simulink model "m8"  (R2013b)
settings: Solver=ode45  StartTime=0.0  StopTime=50  RelTol=1e-3
undefined symbols (not defined in the file): dend, DiscIntNeverNeededParam, Ki, Kp, numd, Tlim, Ts
libraries: powerlib x46, simulink x5, powerlib_extras x3

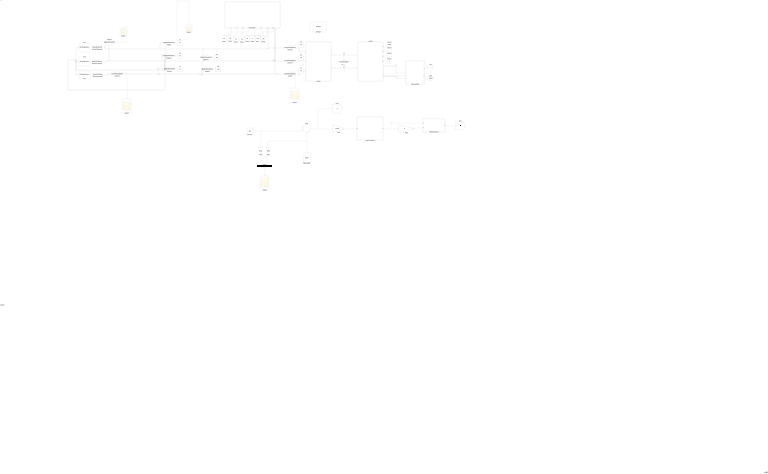
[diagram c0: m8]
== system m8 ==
  AC4 : powerlib/Electrical Sources/AC Voltage Source  Amplitude=400  Phase=0  Frequency=50  SampleTime=0  Measurements=None
  AC5 : powerlib/Electrical Sources/AC Voltage Source  Amplitude=400  Phase=120  Frequency=50  SampleTime=0  Measurements=None
  AC6 : powerlib/Electrical Sources/AC Voltage Source  Amplitude=400  Phase=240  Frequency=50  SampleTime=0  Measurements=None
  Bus Creator : BusCreator  Inputs=2
  C1 : powerlib/Elements/Series RLC Branch  LConnTagsString=__new0  RConnTagsString=__new0  BranchType=C  Resistance=1  Inductance=1e-3  SetiL0=off  InitialCurrent=0  Capacitance=50e-2  Setx0=off  InitialVoltage=0  Measurements=None
  Constant : Constant  Value=146
  Current {,1..3} (4 alike) : powerlib/Measurements/Current Measurement  PhasorSimulation=off  OutputType=Complex  PSBequivalent=0
  Gain3 : Gain  Gain=30/pi
  Gain4 : Gain  Gain=30/pi
  Gain5 : Gain  Gain=8
  Gain6 : Gain  Gain=1/(2*pi)
  Induction Motor : Subsystem
  Integrator : Integrator
  MATLAB Function1 : MATLAB Function  TreatAsAtomicUnit=on
  Mux1 : Mux  Inputs=2
  Scope{1..4,9} (5 alike) : Scope
  Series RLC Branch3 : powerlib/Elements/Series RLC Branch  LConnTagsString=__new0  RConnTagsString=__new0  BranchType=RL  Resistance=0.025  Inductance=80e-6  SetiL0=off  InitialCurrent=0  Capacitance=1e-6  Setx0=off  InitialVoltage=0  Measurements=None
  Series RLC Branch5 : powerlib/Elements/Series RLC Branch  LConnTagsString=__new0  RConnTagsString=__new0  BranchType=RL  Resistance=0.025  Inductance=80e-6  SetiL0=off  InitialCurrent=0  Capacitance=1e-6  Setx0=off  InitialVoltage=0  Measurements=None
  Series RLC Branch7 : powerlib/Elements/Series RLC Branch  LConnTagsString=__new0  RConnTagsString=__new0  BranchType=RL  Resistance=0.025  Inductance=80e-6  SetiL0=off  InitialCurrent=0  Capacitance=1e-6  Setx0=off  InitialVoltage=0  Measurements=None
  Speed controller2 : Subsystem
  Sum4 : Sum  Inputs=|+-
  Voltage {,1..5} (6 alike) : powerlib/Measurements/Voltage Measurement  PhasorSimulation=off  OutputType=Complex  PSBequivalent=0
  inverter : Subsystem
  powergui : powerlib/powergui  Priority=1  SimulationMode=Discrete  SolverType=Tustin  SampleTime=50e-6  frequency=60  SPID=off  DisableSnubberDevices=off  DisableRonSwitches=off  DisableVfSwitches=off  SwTol=0  Interpol=off  DisplayEquations=off  frequencyindice=0  Pbase=100e6  ErrMax=1e-4  Iterations=50  UnitsV=kV  UnitsW=MW  FunctionMessages=off  echomessages=off  HookPort=off  EnableUseOfTLC=off  x0status=blocks  RestoreLinks=warning  ResistiveCurrentMeasurement=off  Frange=[0:2:500]  Ylog=off  Xlog=on  ShowGrid=off  save=off  variable=ZData  structure=ScopeData5  ZoomFFT=off  StartTime=9.8  cycles=1  DisplayStyle=1  fundamental=50  FreqAxis=on  MaxFrequency=1000  frequencyindicesteady=1  RmsSteady=1  display=off  Ts=0  methode=off
  rectifire : Subsystem
  shunt filter : Subsystem
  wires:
  Mux1/1 -> Scope9/1
  [speed] -> inverter/1(speed)
  Sum4/1 -> [e], Gain6/1
  [speed] -> Gain4/1, Sum4/2
  Induction Motor/1(iabc) -> [i]
  Induction Motor/2(speed(rad/s)) -> [speed]
  [i] -> inverter/2(iabc)
  Speed controller2/1(f*) -> Gain5/1, MATLAB Function1/1(f)
  Gain5/1 -> MATLAB Function1/2(v)
  MATLAB Function1/1(Fi) -> [Fi]
  [e] -> inverter/4(e(Te))
  Gain3/1 -> Mux1/1
  Gain4/1 -> Mux1/2
  Gain6/1 -> Speed controller2/1(e)
  [Fi] -> inverter/3(phir*)
  [iLa] -> shunt filter/1(iLa)
  [iLb] -> shunt filter/2(iLb)
  [iLc] -> shunt filter/3(iLc)
  "Voltage "/1 -> Scope1/1, [va]
  Voltage 1/1 -> [vb]
  Voltage 2/1 -> [vc]
  [va] -> shunt filter/4(va)
  [vb] -> shunt filter/5(vb)
  [vc] -> shunt filter/6(vc)
  Voltage 3/1 -> Scope2/1
  [vab] -> shunt filter/7(vab)
  [vcb] -> shunt filter/8(vcb)
  "Current "/1 -> Scope3/1, [iLc]
  Current 2/1 -> [iLa]
  Current 1/1 -> [iLb]
  Voltage 4/1 -> [vab]
  Voltage 5/1 -> [vcb]
  Constant/1 -> Gain3/1, Sum4/1
  Current 3/1 -> Scope4/1
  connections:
  C1/LConn1 -- rectifire/RConn1 -- inverter/RConn1
  C1/RConn1 -- inverter/RConn2 -- rectifire/RConn2
  Voltage 2/LConn2 -- AC5/LConn1 -- AC6/LConn1 -- AC4/LConn1 -- "Voltage "/LConn2 -- Voltage 1/LConn2
  shunt filter/LConn3 -- "Current "/LConn1 -- Voltage 5/LConn1 -- Voltage 2/LConn1 -- Current 3/RConn1
  "Voltage "/LConn1 -- Voltage 3/LConn1 -- Series RLC Branch3/RConn1 -- Voltage 4/LConn1 -- shunt filter/LConn1 -- Current 2/LConn1
  shunt filter/LConn2 -- Current 1/LConn1 -- Voltage 4/LConn2 -- Voltage 5/LConn2 -- Voltage 3/LConn2 -- Series RLC Branch5/RConn1 -- Voltage 1/LConn1
  inverter/LConn1 -- Induction Motor/LConn1
  inverter/LConn2 -- Induction Motor/LConn2
  Series RLC Branch3/LConn1 -- AC4/RConn1
  Series RLC Branch7/LConn1 -- AC6/RConn1
  inverter/LConn3 -- Induction Motor/LConn3
  Series RLC Branch5/LConn1 -- AC5/RConn1
  Current 2/RConn1 -- rectifire/LConn1
  Current 1/RConn1 -- rectifire/LConn2
  "Current "/RConn1 -- rectifire/LConn3
  Series RLC Branch7/RConn1 -- Current 3/LConn1

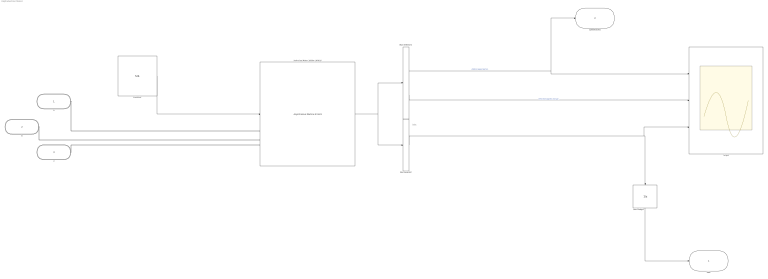
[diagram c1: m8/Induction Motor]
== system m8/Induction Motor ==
  note: iabc
  Bus Selector : BusSelector  OutputSignals=Stator measurements.Stator current is_a (A),Stator measurements.Stator current is_b (A),Stator measurements.Stator current is_c (A)  OutputAsBus=on
  Bus Selector1 : BusSelector  OutputSignals=Mechanical.Rotor speed (wm),Mechanical.Electromagnetic torque Te (N*m)
  Constant : Constant  Value=526
  Induction Motor 100kw / 400 V : powerlib/Machines/Asynchronous Machine SI Units  PresetModel=No  MechanicalLoad=Torque Tm  ShowDetailedParameters=on  RotorType=Squirrel-cage  ReferenceFrame=Rotor  NominalParameters=[ 100e3, 400, 50 ]  Stator=[ 0.087 0.8e-3 ]  Rotor="[ 0.228  0.8e-3 ]"  Cage1=[ 0.022 0.226/377]  Cage2=[ 0.022 0.226/377]  Lm=34.7e-3  Mechanical="[0.3  0.1 2 ]"  PolePairs=2  InitialConditions="[ 1, 0 ,  0 , 0 , 0 , 0 , 0 , 0 ]"  Units=SI  LoadFlowParameters=0  SimulateSaturation=off  Saturation=[0 0;0 0]  TsPowergui=0  TsBlock=-1  IterativeModel=Trapezoidal non iterative  Pmec=0
  Scope : Scope  NumInputPorts=3
  Unit Delay4 : UnitDelay  SampleTime=50e-6
  a : PMIOPort  Port=1  Side=Left
  b : PMIOPort  Port=2  Side=Left
  " c" : PMIOPort  Port=3  Side=Left
  iabc : Outport
  speed(rad/s) : Outport  Port=2
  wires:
  Bus Selector1/1 -> speed(rad/s)/1, Scope/1  "<Rotor speed (wm)>"
  Induction Motor 100kw / 400 V/1 -> Bus Selector1/1, Bus Selector/1
  Bus Selector1/2 -> Scope/2  "<Electromagnetic torque Te (N*m)>"
  Bus Selector/1 -> Unit Delay4/1, Scope/3
  Unit Delay4/1 -> iabc/1
  Constant/1 -> Induction Motor 100kw / 400 V/1
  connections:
  " c"/RConn1 -- Induction Motor 100kw / 400 V/LConn3
  a/RConn1 -- Induction Motor 100kw / 400 V/LConn1
  b/RConn1 -- Induction Motor 100kw / 400 V/LConn2

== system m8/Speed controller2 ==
  e : Inport
  Discrete-Time Integrator : DiscreteIntegrator  IntegratorMethod=Integration: Trapezoidal  SampleTime=Ts  LimitOutput=on  UpperSaturationLimit=Tlim  LowerSaturationLimit=0  ICPrevOutput=DiscIntNeverNeededParam  ICPrevScaledInput=DiscIntNeverNeededParam
  Gain : Gain  Gain=Ki
  Gain1 : Gain  Gain=Kp
  Saturation : Saturate  UpperLimit=Tlim  LowerLimit=0
  Sum2 : Sum
  f* : Outport  InitialOutput=0
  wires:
  Gain1/1 -> Sum2/1
  Gain/1 -> Discrete-Time Integrator/1
  e/1 -> Gain/1, Gain1/1
  Discrete-Time Integrator/1 -> Sum2/2
  Sum2/1 -> Saturation/1
  Saturation/1 -> f*/1

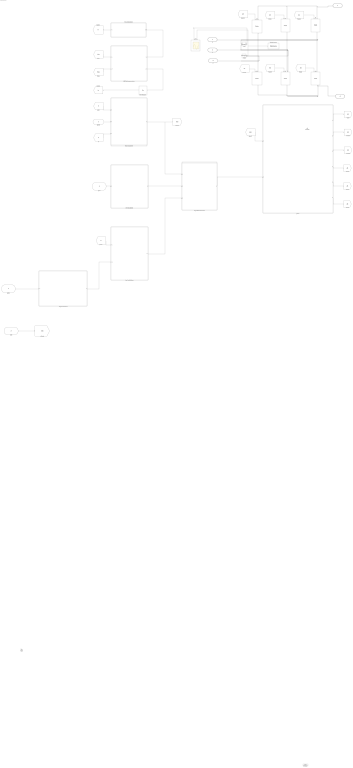
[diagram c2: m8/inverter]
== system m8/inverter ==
  speed : Inport
  iabc : Inport  Port=2
  phir* : Inport  Port=3
  e(Te) : Inport  Port=4
  ABC to dq conversion : Subsystem
  Display : Display
  Flux Calculation : Subsystem
  Gain : Gain
  S{1..6} (6 alike) : powerlib/Power Electronics/IGBT//Diode  Ron=1e-3  Rs=1e5  Cs=inf  Measurements=on
  Teta Calculation : Subsystem
  To Workspace : ToWorkspace  VariableName=VacM  SampleTime=-1  SaveFormat=Timeseries
  Torque controller : Subsystem
  Unit Delay5 : UnitDelay  SampleTime=50e-6
  Vac : powerlib/Measurements/Voltage Measurement  PhasorSimulation=off  OutputType=Complex  PSBequivalent=0
  Vac1 : powerlib/Measurements/Voltage Measurement  PhasorSimulation=off  OutputType=Complex  PSBequivalent=0
  dq to ABC conversion : Subsystem
  id* Calculation : Subsystem
  iqs* calculation : Subsystem
  pwm : Subsystem
  vac : Scope  NumInputPorts=2
  a : PMIOPort  Port=1  Side=Left
  + : PMIOPort  Port=2  Side=Right
  b : PMIOPort  Port=3  Side=Left
  _ : PMIOPort  Port=4  Side=Right
  c : PMIOPort  Port=5  Side=Left
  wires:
  [A5] -> S5/1
  [A3] -> S3/1
  [A1] -> S1/1
  [A2] -> S2/1
  [A6] -> S6/1
  [A4] -> S4/1
  Vac/1 -> vac/1
  Vac1/1 -> To Workspace/1, vac/2
  e(Te)/1 -> Torque controller/1(e)
  dq to ABC conversion/1(Iabc*) -> pwm/2(Iabc*)
  iqs* calculation/1(Iq*) -> dq to ABC conversion/3(Iq*)
  id* Calculation/1(Id*) -> dq to ABC conversion/2(Id*)
  Teta Calculation/1(Teta) -> dq to ABC conversion/1(Teta), [Teta]
  phir*/1 -> id* Calculation/1(Phir*)
  Torque controller/1(Te*) -> iqs* calculation/2(Te*)
  ABC to dq conversion/2(Iq) -> Unit Delay5/1
  ABC to dq conversion/1(Id) -> Flux Calculation/1(Id)
  Flux Calculation/1(Phir) -> [fi]
  [fi] -> Teta Calculation/1(Phir)
  Unit Delay5/1 -> [iq]
  [iq] -> Teta Calculation/3(Iq)
  [fi] -> iqs* calculation/1(Phir)
  [Teta] -> ABC to dq conversion/2(Teta)
  speed/1 -> Teta Calculation/2(wm)
  iabc/1 -> [iabc]
  [iabc] -> ABC to dq conversion/1(Iabc)
  [iabc] -> pwm/1(Iabc)
  pwm/1(s1) -> [A1]
  pwm/2(s2) -> [A2]
  pwm/3(s3) -> [A3]
  pwm/4(s4) -> [A4]
  pwm/5(s5) -> [A5]
  pwm/6(s6) -> [A6]
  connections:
  S4/RConn1 -- _/RConn1 -- S2/RConn1 -- S6/RConn1
  S6/LConn1 -- Vac1/LConn1 -- Vac/LConn2 -- b/RConn1 -- S3/RConn1
  S5/LConn1 -- S3/LConn1 -- +/RConn1 -- S1/LConn1
  S1/RConn1 -- Vac/LConn1 -- a/RConn1 -- S4/LConn1
  S5/RConn1 -- c/RConn1 -- Vac1/LConn2 -- S2/LConn1

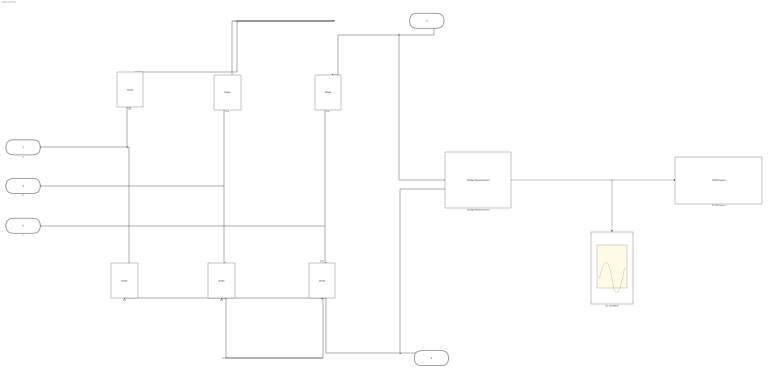
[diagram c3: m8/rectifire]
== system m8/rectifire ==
  D{1..6} (6 alike) : powerlib/Power Electronics/Diode  Ron=0.001  Lon=0  Vf=0.8  IC=0  UseSnubber=off  Rs=500  Cs=250e-9  Measurements=on
  DC VOLTAGE : Scope
  To Workspace : ToWorkspace  VariableName=VDC  SampleTime=-1  SaveFormat=Timeseries
  Voltage Measurement : powerlib/Measurements/Voltage Measurement  PhasorSimulation=off  OutputType=Complex  PSBequivalent=0
  a : PMIOPort  Port=1  Side=Left
  + : PMIOPort  Port=2  Side=Right
  b : PMIOPort  Port=3  Side=Left
  _ : PMIOPort  Port=4  Side=Right
  c : PMIOPort  Port=5  Side=Left
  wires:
  Voltage Measurement/1 -> To Workspace/1, DC VOLTAGE/1
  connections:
  Voltage Measurement/LConn2 -- _/RConn1 -- D6/LConn1 -- D4/LConn1 -- D2/LConn1
  b/RConn1 -- D6/RConn1 -- D3/LConn1
  a/RConn1 -- D4/RConn1 -- D1/LConn1
  Voltage Measurement/LConn1 -- +/RConn1 -- D1/RConn1 -- D3/RConn1 -- D5/RConn1
  c/RConn1 -- D2/RConn1 -- D5/LConn1

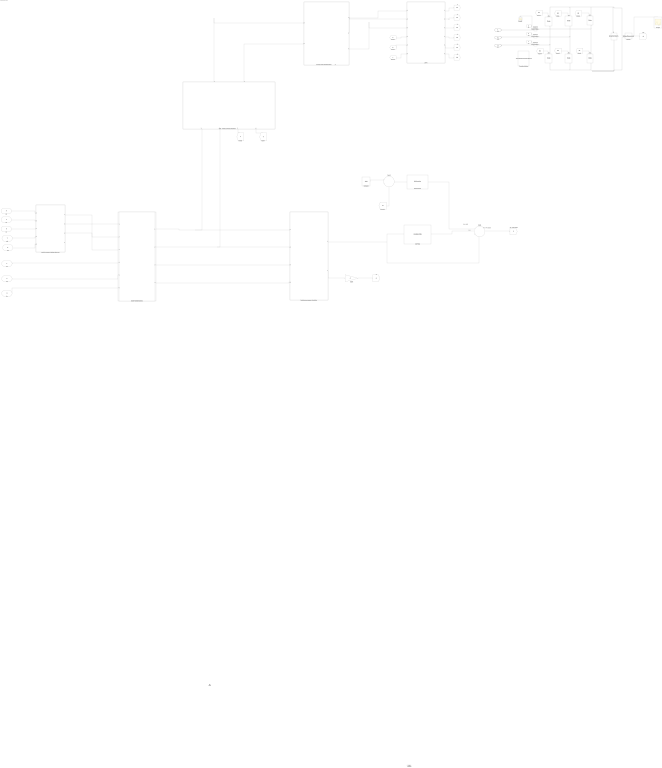
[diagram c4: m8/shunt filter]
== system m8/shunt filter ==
  note: -P(~)+P(-)LOSS
  note: P(-)
  note: P(-) LOSS
  iLa : Inport
  iLb : Inport  Port=2
  iLc : Inport  Port=3
  va : Inport  Port=4
  vb : Inport  Port=5
  vc : Inport  Port=6
  vab : Inport  Port=7
  vcb : Inport  Port=8
  " (alfa -  betta) currents calculation         " : Subsystem
  " Inverse clarke Transformation           1" : Subsystem
  2nd Filter : powerlib_extras/Control  Blocks/2nd-Order Filter  FilterType=Lowpass  Fo=50  Zeta=0.707  Initialize=off  Vac_Init=[1 45 60]  Vdc_Init=-0.5  PlotResponse=off  param1=[1 500 1]
  C : powerlib/Elements/Series RLC Branch  LConnTagsString=__new0  RConnTagsString=__new0  BranchType=C  Resistance=1  Inductance=1e-3  SetiL0=off  InitialCurrent=0  Capacitance=.045  Setx0=on  InitialVoltage=1000  Measurements=None
  Clarke Transformation1 : Subsystem
  Constant : Constant  Value=1000
  Coupling Inductor : powerlib/Elements/Three-Phase Series RLC Branch  LConnTagsString=A|B|C  RConnTagsString=A|B|C  BranchType=RL  Resistance=0.9  Inductance=0.001  Capacitance=1e-6  Measurements=None
  Current 1 : powerlib/Measurements/Current Measurement  PhasorSimulation=off  OutputType=Complex  PSBequivalent=0
  Current 2 : powerlib/Measurements/Current Measurement  PhasorSimulation=off  OutputType=Complex  PSBequivalent=0
  Current 3 : powerlib/Measurements/Current Measurement  PhasorSimulation=off  OutputType=Complex  PSBequivalent=0
  Display : Display
  Gain : Gain
  Gain6 : Gain  Gain=-1
  "Instantaneous power calculation " : Subsystem
  PID Controller : simulink/Continuous/PID Controller  Controller=PI  TimeDomain=Discrete-time  SampleTime=50e-6  IntegratorMethod=Forward Euler  FilterMethod=Forward Euler  Form=Parallel  P=400  I=100  D=0  N=100  InitialConditionSource=internal  InitialConditionForIntegrator=0  InitialConditionForFilter=0  ExternalReset=none  LimitOutput=off  UpperSaturationLimit=inf  LowerSaturationLimit=-inf  LinearizeAsGain=on  AntiWindupMode=none  Kb=1  TrackingMode=off  Kt=1  PParamMin=[]  PParamMax=[]  IParamMin=[]  IParamMax=[]  DParamMin=[]  DParamMax=[]  NParamMin=[]  NParamMax=[]  KbParamMin=[]  KbParamMax=[]  KtParamMin=[]  KtParamMax=[]  POutMin=[]  POutMax=[]  IOutMin=[]  IOutMax=[]  DOutMin=[]  DOutMax=[]  NOutMin=[]  NOutMax=[]  KbOutMin=[]  KbOutMax=[]  KtOutMin=[]  KtOutMax=[]  IntegratorOutMin=[]  IntegratorOutMax=[]  FilterOutMin=[]  FilterOutMax=[]  SumOutMin=[]  SumOutMax=[]  SumI1OutMin=[]  SumI1OutMax=[]  SumI2OutMin=[]  SumI2OutMax=[]  SumI3OutMin=[]  SumI3OutMax=[]  SumDOutMin=[]  SumDOutMax=[]  SaturationOutMin=[]  SaturationOutMax=[]  IntegratorContinuousStateAttributes=''  IntegratorStateMustResolveToSignalObject=off  IntegratorRTWStateStorageClass=Auto  FilterContinuousStateAttributes=''  FilterStateMustResolveToSignalObject=off  FilterRTWStateStorageClass=Auto
  S{1..6} (6 alike) : powerlib/Power Electronics/IGBT//Diode  Ron=1e-3  Rs=1e5  Cs=inf  Measurements=on
  Scope1 : Scope
  Scope3 : Scope
  Sum1 : Sum  Inputs=|+-
  Sum4 : Sum  Inputs=|++-
  "Voltage " : powerlib/Measurements/Voltage Measurement  PhasorSimulation=off  OutputType=Complex  PSBequivalent=0
  positive sequence Voltage Detector : Subsystem
  pwm : Subsystem
  ica : PMIOPort  Port=1  Side=Left
  icb : PMIOPort  Port=2  Side=Left
  icc : PMIOPort  Port=3  Side=Left
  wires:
  [B5] -> S5/1
  [B3] -> S3/1
  [B1] -> S1/1
  [B2] -> S2/1
  [B6] -> S6/1
  [B4] -> S4/1
  iLa/1 -> Clarke Transformation1/4(iLa)
  iLb/1 -> Clarke Transformation1/5(iLb)
  iLc/1 -> Clarke Transformation1/6(iLc)
  Clarke Transformation1/1(v alfa') -> "Instantaneous power calculation "/1(v alfa'), " (alfa -  betta) currents calculation         "/1(v alfa')
  Clarke Transformation1/2(v betta') -> "Instantaneous power calculation "/2(v betta'), " (alfa -  betta) currents calculation         "/2(v betta')
  Clarke Transformation1/3(i alfa) -> "Instantaneous power calculation "/3(i alfa)
  Clarke Transformation1/4(i betta) -> "Instantaneous power calculation "/4(i betta)
  " (alfa -  betta) currents calculation         "/1(ic alfa*) -> " Inverse clarke Transformation           1"/1(ic alfa*)
  " (alfa -  betta) currents calculation         "/2(ic betta*) -> " Inverse clarke Transformation           1"/2(ic betta*)
  "Instantaneous power calculation "/1(p) -> 2nd Filter/1, Sum4/3
  2nd Filter/1 -> Sum4/2
  PID Controller/1 -> Sum4/1
  Sum1/1 -> PID Controller/1
  Sum4/1 -> [P]
  "Instantaneous power calculation "/2(q) -> Gain6/1
  Gain6/1 -> [q]
  [P] -> " (alfa -  betta) currents calculation         "/3(-p(~)+P(-)LOSS)
  [q] -> " (alfa -  betta) currents calculation         "/4(-q)
  Current 1/1 -> [b]
  Current 2/1 -> Scope1/1, [a]
  Current 3/1 -> [c]
  [a] -> pwm/4(Ica)
  [b] -> pwm/5(Icb)
  [c] -> pwm/6(Icc)
  " Inverse clarke Transformation           1"/1(ica*) -> pwm/1(Ica*)
  " Inverse clarke Transformation           1"/2(icb*) -> pwm/2(Icb*)
  " Inverse clarke Transformation           1"/3(icc*) -> pwm/3(Icc*)
  pwm/1(s1) -> [B1]
  pwm/2(s2) -> [B2]
  pwm/3(s3) -> [B3]
  pwm/4(s4) -> [B4]
  pwm/5(s5) -> [B5]
  pwm/6(s6) -> [B6]
  "Voltage "/1 -> Scope3/1, [vd]
  [vd] -> Sum1/2
  Constant/1 -> Sum1/1
  va/1 -> positive sequence Voltage Detector/1(va)
  vb/1 -> positive sequence Voltage Detector/2(vb)
  vc/1 -> positive sequence Voltage Detector/3(vc)
  vab/1 -> positive sequence Voltage Detector/4(vab)
  vcb/1 -> positive sequence Voltage Detector/5(vcb)
  positive sequence Voltage Detector/1(va') -> Clarke Transformation1/1(va')
  positive sequence Voltage Detector/2(vb') -> Clarke Transformation1/2(vb')
  positive sequence Voltage Detector/3(vc') -> Clarke Transformation1/3(vc')
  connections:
  S2/RConn1 -- S6/RConn1 -- C/RConn1 -- "Voltage "/LConn2 -- S4/RConn1
  S3/RConn1 -- Current 1/LConn1 -- S6/LConn1
  S5/LConn1 -- S3/LConn1 -- C/LConn1 -- "Voltage "/LConn1 -- S1/LConn1
  S1/RConn1 -- S4/LConn1 -- Current 2/LConn1
  S5/RConn1 -- Current 3/LConn1 -- S2/LConn1
  ica/RConn1 -- Current 2/RConn1
  icb/RConn1 -- Current 1/RConn1
  icc/RConn1 -- Current 3/RConn1

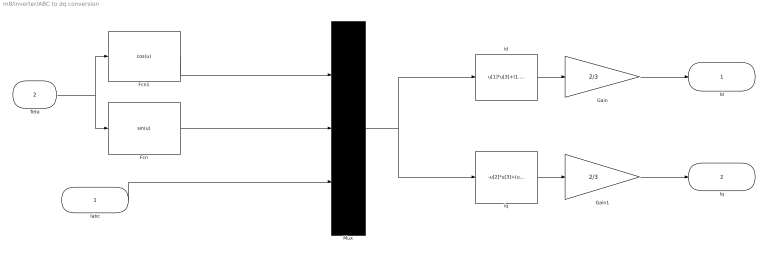
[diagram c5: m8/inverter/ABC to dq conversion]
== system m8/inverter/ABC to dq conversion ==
  Iabc : Inport
  Teta : Inport  Port=2
  Fcn : Fcn  Expr=sin(u)
  Fcn1 : Fcn  Expr=cos(u)
  Gain : Gain  Gain=2/3
  Gain1 : Gain  Gain=2/3
  Mux : Mux  Inputs=[1 1 3]
  id : Fcn  Expr=u[1]*u[3]+(1.7320508*u[2]-u[1])*u[4]*0.5+(-u[1]-1.7320508*u[2])*u[5]*0.5
  iq : Fcn  Expr=-u[2]*u[3]+(u[2]+1.7320508*u[1])*u[4]*0.5+(u[2]-1.7320508*u[1])*u[5]*0.5
  Id : Outport  InitialOutput=0
  Iq : Outport  Port=2  InitialOutput=0
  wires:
  Fcn/1 -> Mux/2
  Fcn1/1 -> Mux/1
  Teta/1 -> Fcn1/1, Fcn/1
  Mux/1 -> id/1, iq/1
  Iabc/1 -> Mux/3
  iq/1 -> Gain1/1
  id/1 -> Gain/1
  Gain/1 -> Id/1
  Gain1/1 -> Iq/1

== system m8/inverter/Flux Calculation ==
  note: Phir = Lm *Id / (1 +Tr .s)
  note: Lm = 34.7 mH
  note: Lr = Ll'r +Lm = 0.8 +34.7= 35.5 mH
  note: Tr = Lr / Rr = 0.1557 s
  note: Rr = 0.228 ohms
  Id : Inport
  Discrete Tranfer Function : Subsystem
  Lm : Gain  Gain=34.7e-3
  Phir : Outport
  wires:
  Discrete Tranfer Function/1(Out) -> Phir/1
  Id/1 -> Lm/1
  Lm/1 -> Discrete Tranfer Function/1(In)

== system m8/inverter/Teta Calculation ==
  note: Teta= Electrical angle= integ ( wr + wm)
  note: wr = Rotor frequency (rad/s) = Lm *Iq / ( Tr * Phir)
  note: Lm = 34.7 mH
  note: Rr= 0.228 ohms
  note: Lr = Ll'r +Lm = 0.8 +34.7= 35.5 mH
  note: wm= Rotor mechanical speed (rad/s)
  note: Tr = Lr / Rr = 0.1557 s
  Phir : Inport
  wm : Inport  Port=2
  Iq : Inport  Port=3
  Discrete-Time Integrator : DiscreteIntegrator  SampleTime=50e-6  ICPrevOutput=DiscIntNeverNeededParam  ICPrevScaledInput=DiscIntNeverNeededParam
  Fcn : Fcn  Expr=34.7e-3*u[1]/(u[2]*0.1557+1e-3)
  Gain2 : Gain
  Gain3 : Gain  Gain=2
  Mux : Mux  Inputs=2
  Sum : Sum
  Teta : Outport  InitialOutput=0
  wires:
  Discrete-Time Integrator/1 -> Teta/1
  Sum/1 -> Discrete-Time Integrator/1
  Gain3/1 -> Sum/2
  Gain2/1 -> Sum/1
  wm/1 -> Gain3/1
  Fcn/1 -> Gain2/1
  Phir/1 -> Mux/2
  Iq/1 -> Mux/1
  Mux/1 -> Fcn/1

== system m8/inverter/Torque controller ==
  e : Inport
  Discrete-Time Integrator : DiscreteIntegrator  IntegratorMethod=Integration: Trapezoidal  SampleTime=Ts  LimitOutput=on  UpperSaturationLimit=Tlim  LowerSaturationLimit=0  ICPrevOutput=DiscIntNeverNeededParam  ICPrevScaledInput=DiscIntNeverNeededParam
  Gain : Gain  Gain=Ki
  Gain1 : Gain  Gain=Kp
  Saturation : Saturate  UpperLimit=Tlim  LowerLimit=0
  Sum2 : Sum
  Te* : Outport  InitialOutput=0
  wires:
  Gain1/1 -> Sum2/1
  Gain/1 -> Discrete-Time Integrator/1
  e/1 -> Gain1/1, Gain/1
  Discrete-Time Integrator/1 -> Sum2/2
  Sum2/1 -> Saturation/1
  Saturation/1 -> Te*/1

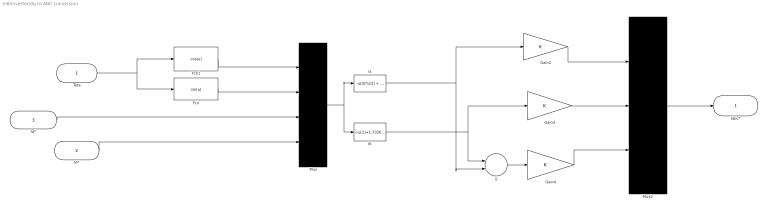
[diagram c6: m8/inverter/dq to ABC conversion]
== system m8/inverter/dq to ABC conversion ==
  Teta : Inport
  Id* : Inport  Port=2
  Iq* : Inport  Port=3
  Fcn : Fcn  Expr=sin(u)
  Fcn1 : Fcn  Expr=cos(u)
  Gain2 : Gain
  Gain3 : Gain
  Gain4 : Gain
  Mux : Mux
  Mux2 : Mux  Inputs=3
  ia : Fcn  Expr=-u[3]*u[2] + u[4]*u[1]
  ib : Fcn  Expr=(-u[1]+1.7320508*u[2])*u[4]*0.5+(u[2]+1.7320508*u[1])*u[3]*0.5
  ic : Sum  Inputs=--
  Iabc* : Outport  InitialOutput=0
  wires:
  Fcn/1 -> Mux/2
  Fcn1/1 -> Mux/1
  Mux2/1 -> Iabc*/1
  Mux/1 -> ia/1, ib/1
  Teta/1 -> Fcn/1, Fcn1/1
  Iq*/1 -> Mux/3
  Id*/1 -> Mux/4
  Gain3/1 -> Mux2/2
  ic/1 -> Gain4/1
  Gain4/1 -> Mux2/3
  Gain2/1 -> Mux2/1
  ia/1 -> Gain2/1, ic/2
  ib/1 -> Gain3/1, ic/1

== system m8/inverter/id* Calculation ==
  note: Id* = Phir*/ Lm
  note: Lm= 34.7 mH
  Phir* : Inport
  KF : Gain  Gain=1/34.7e-3
  Id* : Outport
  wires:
  KF/1 -> Id*/1
  Phir*/1 -> KF/1

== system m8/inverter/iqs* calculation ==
  note: Iq= ( 2/3) * (2/p) * ( Lr/Lm) * (Te / Phir)
  note: Lm = 34.7 mH
  note: Lr = Ll'r +Lm = 0.8 +34.7= 35.5 mH
  note: p= nb of poles = 4
  note: Iq= 0.341 * (Te / Phir)
  Phir : Inport
  Te* : Inport  Port=2
  Fcn : Fcn  Expr=u[1]*0.341/(u[2]+1e-3)
  Mux1 : Mux  Inputs=2
  Iq* : Outport  InitialOutput=0
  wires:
  Phir/1 -> Mux1/2
  Fcn/1 -> Iq*/1
  Te*/1 -> Mux1/1
  Mux1/1 -> Fcn/1

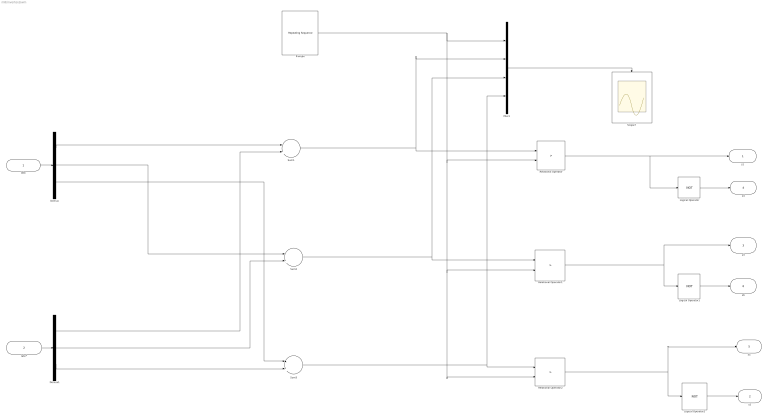
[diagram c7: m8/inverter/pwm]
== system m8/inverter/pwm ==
  Iabc : Inport
  Iabc* : Inport  Port=2
  Demux : Demux  Outputs=3
  Demux1 : Demux  Outputs=3
  Logical Operator : Logic  Operator=NOT
  Logical Operator1 : Logic  Operator=NOT
  Logical Operator2 : Logic  Operator=NOT
  Mux1 : Mux
  Relational Operator : RelationalOperator  Operator=>  OutDataTypeStr=boolean
  Relational Operator1 : RelationalOperator  Operator=>  OutDataTypeStr=boolean
  Relational Operator2 : RelationalOperator  Operator=>  OutDataTypeStr=boolean
  Scope7 : Scope
  Sum1 : Sum  Inputs=-+
  Sum2 : Sum  Inputs=-+
  Sum3 : Sum  Inputs=-+
  Traingle : simulink/Sources/Repeating Sequence  rep_seq_t=[0 1/2000/4 3/2000/4 1/2000]  rep_seq_y=[0 -30 30 0]
  s1 : Outport
  s2 : Outport  Port=2
  s3 : Outport  Port=3
  s4 : Outport  Port=4
  s5 : Outport  Port=5
  s6 : Outport  Port=6
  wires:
  Demux/1 -> Sum1/1
  Demux1/1 -> Sum1/2
  Demux/2 -> Sum2/1
  Demux1/2 -> Sum2/2
  Demux/3 -> Sum3/1
  Demux1/3 -> Sum3/2
  Relational Operator/1 -> Logical Operator/1, s1/1
  Logical Operator/1 -> s4/1
  Relational Operator1/1 -> s3/1, Logical Operator1/1
  Logical Operator1/1 -> s6/1
  Relational Operator2/1 -> s5/1, Logical Operator2/1
  Logical Operator2/1 -> s2/1
  Sum1/1 -> Relational Operator/1, Mux1/2
  Sum2/1 -> Mux1/3, Relational Operator1/1
  Sum3/1 -> Mux1/4, Relational Operator2/1
  Traingle/1 -> Mux1/1, Relational Operator/2, Relational Operator1/2, Relational Operator2/2
  Mux1/1 -> Scope7/1
  Iabc/1 -> Demux/1
  Iabc*/1 -> Demux1/1

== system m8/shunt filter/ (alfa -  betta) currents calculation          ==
  v alfa' : Inport
  v betta' : Inport  Port=2
  -p(~)+P(-)LOSS : Inport  Port=3
  -q : Inport  Port=4
  Fcn : Fcn  Expr=(1/(u[1]^2+u[2]^2))*((u[1]*u[3])+(u[2]*u[4]))
  Fcn1 : Fcn  Expr=(1/(u[1]^2+u[2]^2))*((u[2]*u[3])-(u[1]*u[4]))
  Mux : Mux
  ic alfa* : Outport  InitialOutput=0
  ic betta* : Outport  Port=2  InitialOutput=0
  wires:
  v alfa'/1 -> Mux/1
  v betta'/1 -> Mux/2
  -p(~)+P(-)LOSS/1 -> Mux/3
  -q/1 -> Mux/4
  Mux/1 -> Fcn/1, Fcn1/1
  Fcn/1 -> ic alfa*/1
  Fcn1/1 -> ic betta*/1

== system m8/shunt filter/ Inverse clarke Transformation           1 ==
  ic alfa* : Inport
  ic betta* : Inport  Port=2
  Fcn : Fcn  Expr=sqrt(2/3)*u[1]
  Fcn1 : Fcn  Expr=sqrt(2/3)*((-u[1]/2)+((sqrt(3)/2)*u[2]))
  Fcn2 : Fcn  Expr=sqrt(2/3)*((-u[1]/2)-((sqrt(3)/2)*u[2]))
  Mux : Mux  Inputs=2
  ica* : Outport  InitialOutput=0
  icb* : Outport  Port=2  InitialOutput=0
  icc* : Outport  Port=3  InitialOutput=0
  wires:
  ic betta*/1 -> Mux/2
  ic alfa*/1 -> Mux/1
  Mux/1 -> Fcn/1, Fcn2/1, Fcn1/1
  Fcn/1 -> ica*/1
  Fcn1/1 -> icb*/1
  Fcn2/1 -> icc*/1

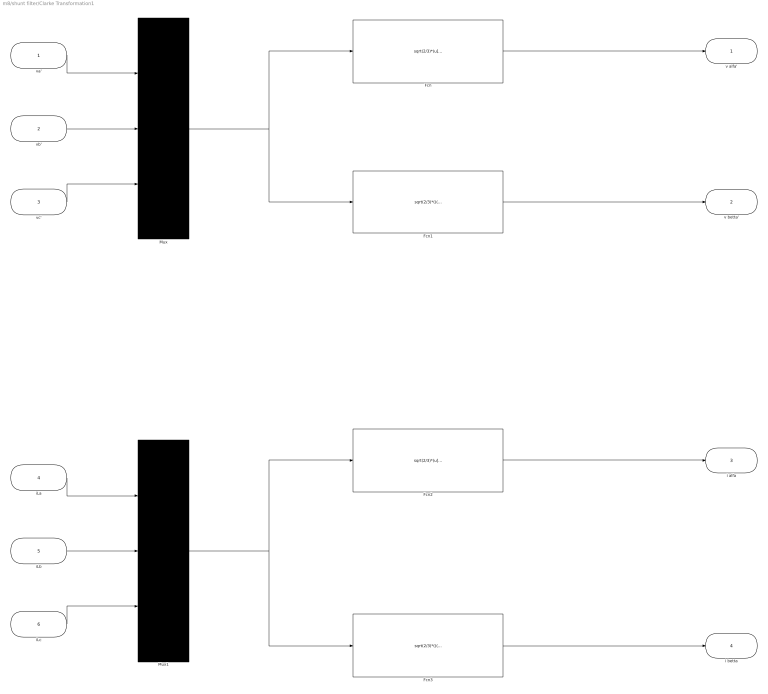
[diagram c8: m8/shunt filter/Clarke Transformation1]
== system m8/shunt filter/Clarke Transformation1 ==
  va' : Inport
  vb' : Inport  Port=2
  vc' : Inport  Port=3
  iLa : Inport  Port=4
  iLb : Inport  Port=5
  iLc : Inport  Port=6
  Fcn : Fcn  Expr=sqrt(2/3)*(u[1]-(u[2]/2)-(u[3]/2))
  Fcn1 : Fcn  Expr=sqrt(2/3)*(((sqrt(3)/2)*u[2])-((sqrt(3)/2)*u[3]))
  Fcn2 : Fcn  Expr=sqrt(2/3)*(u[1]-(u[2]/2)-(u[3]/2))
  Fcn3 : Fcn  Expr=sqrt(2/3)*(((sqrt(3)/2)*u[2])-((sqrt(3)/2)*u[3]))
  Mux : Mux  Inputs=3
  Mux1 : Mux  Inputs=3
  v alfa' : Outport  InitialOutput=0
  v betta' : Outport  Port=2  InitialOutput=0
  i alfa : Outport  Port=3  InitialOutput=0
  i betta : Outport  Port=4  InitialOutput=0
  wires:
  va'/1 -> Mux/1
  vb'/1 -> Mux/2
  vc'/1 -> Mux/3
  Fcn/1 -> v alfa'/1
  Fcn1/1 -> v betta'/1
  Mux/1 -> Fcn/1, Fcn1/1
  iLa/1 -> Mux1/1
  iLb/1 -> Mux1/2
  iLc/1 -> Mux1/3
  Mux1/1 -> Fcn2/1, Fcn3/1
  Fcn2/1 -> i alfa/1
  Fcn3/1 -> i betta/1

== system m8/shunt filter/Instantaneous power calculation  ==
  v alfa' : Inport
  v betta' : Inport  Port=2
  i alfa : Inport  Port=3
  i betta : Inport  Port=4
  Fcn : Fcn  Expr=(u[1]*u[3])+(u[2]*u[4])
  Fcn1 : Fcn  Expr=(u[2]*u[3])-(u[1]*u[4])
  Mux : Mux
  p : Outport  InitialOutput=0
  q : Outport  Port=2  InitialOutput=0
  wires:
  Mux/1 -> Fcn/1, Fcn1/1
  v alfa'/1 -> Mux/1
  v betta'/1 -> Mux/2
  i alfa/1 -> Mux/3
  i betta/1 -> Mux/4
  Fcn/1 -> p/1
  Fcn1/1 -> q/1

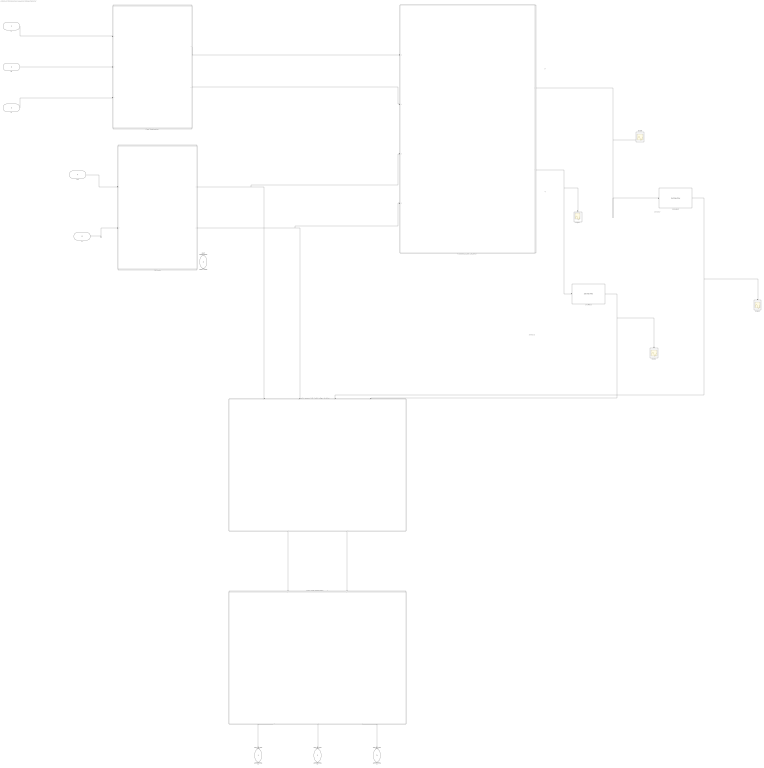
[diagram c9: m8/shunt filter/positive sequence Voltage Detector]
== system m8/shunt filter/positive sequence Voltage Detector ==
  note: average p'
  note: average q'
  note: p'
  note: q'
  va : Inport
  vb : Inport  Port=2
  vc : Inport  Port=3
  vab : Inport  Port=4
  vcb : Inport  Port=5
  " Inverse clarke Transformation           1" : Subsystem
  " positive sequence (alfa -  betta) voltage calculation           " : Subsystem
  2nd Filter1 : powerlib_extras/Control  Blocks/2nd-Order Filter  FilterType=Lowpass  Fo=50  Zeta=1  Initialize=off  Vac_Init=[1 45 60]  Vdc_Init=-0.5  PlotResponse=off  param1=[1 500 1]
  2nd Filter2 : powerlib_extras/Control  Blocks/2nd-Order Filter  FilterType=Lowpass  Fo=50  Zeta=1  Initialize=off  Vac_Init=[1 45 60]  Vdc_Init=-0.5  PlotResponse=off  param1=[1 500 1]
  Clarke Transformation : Subsystem
  "Instantaneous power calculation " : Subsystem
  PLL Circute : Subsystem
  Scope{1,4..6} (4 alike) : Scope
  va' : Outport  InitialOutput=0
  vb' : Outport  Port=2  InitialOutput=0
  vc' : Outport  Port=3  InitialOutput=0
  asad : Outport  Port=4  InitialOutput=0
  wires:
  va/1 -> Clarke Transformation/1(va)
  vc/1 -> Clarke Transformation/3(vc)
  "Instantaneous power calculation "/1(p') -> Scope6/1, 2nd Filter2/1
  "Instantaneous power calculation "/2(q') -> Scope4/1, 2nd Filter1/1
  Clarke Transformation/1(v alfa) -> "Instantaneous power calculation "/1(v alfa)
  Clarke Transformation/2(v betta) -> "Instantaneous power calculation "/2(v betta)
  PLL Circute/1(i alfa') -> "Instantaneous power calculation "/3(i alfa'), " positive sequence (alfa -  betta) voltage calculation           "/1(i alfa')
  PLL Circute/2(i beta') -> "Instantaneous power calculation "/4(i betta'), " positive sequence (alfa -  betta) voltage calculation           "/2(i betta')
  " positive sequence (alfa -  betta) voltage calculation           "/1(v alfa') -> " Inverse clarke Transformation           1"/1(v alfa')
  " positive sequence (alfa -  betta) voltage calculation           "/2(v betta') -> " Inverse clarke Transformation           1"/2(v betta')
  " Inverse clarke Transformation           1"/1(va') -> va'/1
  " Inverse clarke Transformation           1"/2(vb') -> vb'/1
  " Inverse clarke Transformation           1"/3(vc') -> vc'/1
  2nd Filter2/1 -> Scope5/1, " positive sequence (alfa -  betta) voltage calculation           "/3(p(-)')
  2nd Filter1/1 -> Scope1/1, " positive sequence (alfa -  betta) voltage calculation           "/4(q(-)')
  vb/1 -> Clarke Transformation/2(vb)
  vab/1 -> PLL Circute/1(vab)
  vcb/1 -> PLL Circute/2(vcb)

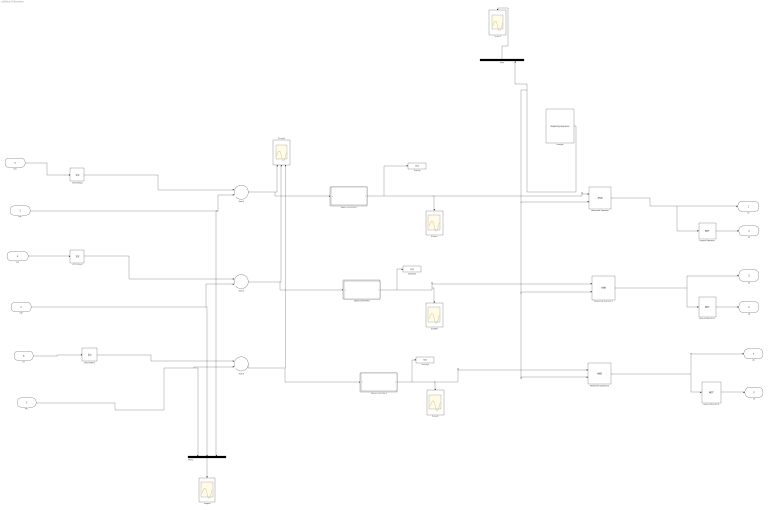
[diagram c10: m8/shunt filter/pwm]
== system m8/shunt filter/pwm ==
  Ica* : Inport
  Icb* : Inport  Port=2
  Icc* : Inport  Port=3
  Ica : Inport  Port=4
  Icb : Inport  Port=5
  Icc : Inport  Port=6
  Display : Display
  Display1 : Display
  Display2 : Display
  Logical Operator : Logic  Operator=NOT
  Logical Operator1 : Logic  Operator=NOT
  Logical Operator2 : Logic  Operator=NOT
  Mux : Mux
  Mux2 : Mux  Inputs=3
  Relational Operator : RelationalOperator  OutDataTypeStr=boolean  SampleTime=50e-6
  Relational Operator1 : RelationalOperator  OutDataTypeStr=boolean  SampleTime=50e-6
  Relational Operator2 : RelationalOperator  OutDataTypeStr=boolean  SampleTime=50e-6
  Scope{2,4..7} (5 alike) : Scope
  Scope8 : Scope  NumInputPorts=3
  Speed controller1 : Subsystem
  Speed controller2 : Subsystem
  Speed controller3 : Subsystem
  Sum1 : Sum  Inputs=-+
  Sum2 : Sum  Inputs=-+
  Sum3 : Sum  Inputs=-+
  Traingle : simulink/Sources/Repeating Sequence  rep_seq_t=[0 1/10000/4 3/10000/4 1/10000]  rep_seq_y=[0 -100 100 0]
  Unit Delay1 : UnitDelay  SampleTime=-1
  Unit Delay2 : UnitDelay  SampleTime=-1
  Unit Delay3 : UnitDelay  SampleTime=-1
  s1 : Outport
  s2 : Outport  Port=2
  s3 : Outport  Port=3
  s4 : Outport  Port=4
  s5 : Outport  Port=5
  s6 : Outport  Port=6
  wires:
  Relational Operator/1 -> Logical Operator/1, s1/1
  Logical Operator/1 -> s4/1
  Relational Operator1/1 -> Logical Operator1/1, s3/1
  Logical Operator1/1 -> s6/1
  Relational Operator2/1 -> s5/1, Logical Operator2/1
  Logical Operator2/1 -> s2/1
  Traingle/1 -> Mux/4, Relational Operator2/2, Relational Operator1/2, Relational Operator/2
  Mux/1 -> Scope2/1
  Mux2/1 -> Scope4/1
  Sum3/1 -> Scope8/3, Speed controller3/1(e)
  Sum2/1 -> Scope8/2, Speed controller1/1(e)
  Icb/1 -> Unit Delay1/1
  Unit Delay1/1 -> Sum2/1
  Ica*/1 -> Sum1/2, Mux2/3
  Icb*/1 -> Sum2/2, Mux2/2
  Icc*/1 -> Mux2/1, Sum3/2
  Sum1/1 -> Scope8/1, Speed controller2/1(e)
  Speed controller2/1(f*) -> Display/1, Relational Operator/1, Scope7/1
  Speed controller1/1(f*) -> Display1/1, Scope6/1, Relational Operator1/1
  Speed controller3/1(f*) -> Display2/1, Scope5/1, Relational Operator2/1
  Icc/1 -> Unit Delay3/1
  Unit Delay3/1 -> Sum3/1
  Ica/1 -> Unit Delay2/1
  Unit Delay2/1 -> Sum1/1

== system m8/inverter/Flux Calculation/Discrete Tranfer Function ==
  In : Inport
  Discrete Transfer Fcn : DiscreteTransferFcn  Numerator=numd  Denominator=dend  SampleTime=Ts
  Out : Outport  InitialOutput=0
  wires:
  Discrete Transfer Fcn/1 -> Out/1
  In/1 -> Discrete Transfer Fcn/1

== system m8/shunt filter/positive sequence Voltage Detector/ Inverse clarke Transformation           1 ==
  v alfa' : Inport
  v betta' : Inport  Port=2
  Fcn : Fcn  Expr=sqrt(2/3)*u[1]
  Fcn1 : Fcn  Expr=sqrt(2/3)*((-u[1]/2)+((sqrt(3)/2)*u[2]))
  Fcn2 : Fcn  Expr=sqrt(2/3)*((-u[1]/2)-((sqrt(3)/2)*u[2]))
  Mux : Mux  Inputs=2
  va' : Outport  InitialOutput=0
  vb' : Outport  Port=2  InitialOutput=0
  vc' : Outport  Port=3  InitialOutput=0
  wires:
  Mux/1 -> Fcn/1, Fcn2/1, Fcn1/1
  Fcn/1 -> va'/1
  Fcn1/1 -> vb'/1
  Fcn2/1 -> vc'/1
  v alfa'/1 -> Mux/1
  v betta'/1 -> Mux/2

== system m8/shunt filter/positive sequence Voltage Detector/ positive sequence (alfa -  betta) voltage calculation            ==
  i alfa' : Inport
  i betta' : Inport  Port=2
  p(-)' : Inport  Port=3
  q(-)' : Inport  Port=4
  Fcn : Fcn  Expr=(1/(u[1]^2+u[2]^2))*((u[1]*u[3])-(u[2]*u[4]))
  Fcn1 : Fcn  Expr=(1/(u[1]^2+u[2]^2))*((u[2]*u[3])+(u[1]*u[4]))
  Mux : Mux
  v alfa' : Outport  InitialOutput=0
  v betta' : Outport  Port=2  InitialOutput=0
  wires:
  i alfa'/1 -> Mux/1
  i betta'/1 -> Mux/2
  p(-)'/1 -> Mux/3
  q(-)'/1 -> Mux/4
  Mux/1 -> Fcn/1, Fcn1/1
  Fcn/1 -> v alfa'/1
  Fcn1/1 -> v betta'/1

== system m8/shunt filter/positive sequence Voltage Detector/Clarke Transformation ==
  va : Inport
  vb : Inport  Port=2
  vc : Inport  Port=3
  Fcn : Fcn  Expr=sqrt(2/3)*(u[1]-(u[2]/2)-(u[3]/2))
  Fcn1 : Fcn  Expr=sqrt(2/3)*(((sqrt(3)/2)*u[2])-((sqrt(3)/2)*u[3]))
  Mux : Mux  Inputs=3
  v alfa : Outport  InitialOutput=0
  v betta : Outport  Port=2  InitialOutput=0
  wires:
  Fcn/1 -> v alfa/1
  Fcn1/1 -> v betta/1
  Mux/1 -> Fcn/1, Fcn1/1
  va/1 -> Mux/1
  vb/1 -> Mux/2
  vc/1 -> Mux/3

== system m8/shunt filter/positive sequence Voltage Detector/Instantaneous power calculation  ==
  v alfa : Inport
  v betta : Inport  Port=2
  i alfa' : Inport  Port=3
  i betta' : Inport  Port=4
  Fcn : Fcn  Expr=(u[1]*u[3])+(u[2]*u[4])
  Fcn1 : Fcn  Expr=(u[2]*u[3])-(u[1]*u[4])
  Mux : Mux
  p' : Outport  InitialOutput=0
  q' : Outport  Port=2  InitialOutput=0
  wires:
  Mux/1 -> Fcn/1, Fcn1/1
  Fcn1/1 -> q'/1
  Fcn/1 -> p'/1
  v alfa/1 -> Mux/1
  v betta/1 -> Mux/2
  i alfa'/1 -> Mux/3
  i betta'/1 -> Mux/4

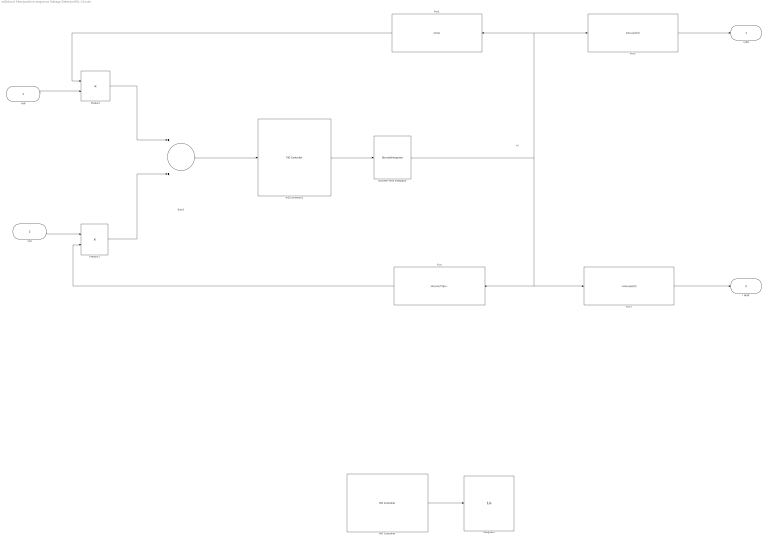
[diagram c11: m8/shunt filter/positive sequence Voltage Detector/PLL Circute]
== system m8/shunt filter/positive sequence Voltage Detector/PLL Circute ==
  note: wt
  vab : Inport
  vcb : Inport  Port=2
  Discrete-Time Integrator : DiscreteIntegrator  IntegratorMethod=Integration: Backward Euler  gainval=.01  SampleTime=50e-6  ICPrevOutput=DiscIntNeverNeededParam  ICPrevScaledInput=DiscIntNeverNeededParam
  Fcn : Fcn  Expr=sin(u+(2*(pi/3)))
  Fcn1 : Fcn  Expr=sin(u)
  Fcn2 : Fcn  Expr=sin(u-(pi/2))
  Fcn3 : Fcn  Expr=-cos(u-(pi/2))
  Integrator : Integrator
  PID Controller : simulink/Continuous/PID Controller  Controller=PI  TimeDomain=Continuous-time  SampleTime=1  IntegratorMethod=Forward Euler  FilterMethod=Forward Euler  Form=Ideal  P=100  I=400  D=0  N=100  InitialConditionSource=internal  InitialConditionForIntegrator=0  InitialConditionForFilter=0  ExternalReset=none  LimitOutput=off  UpperSaturationLimit=inf  LowerSaturationLimit=-inf  LinearizeAsGain=on  AntiWindupMode=none  Kb=1  TrackingMode=off  Kt=1  PParamMin=[]  PParamMax=[]  IParamMin=[]  IParamMax=[]  DParamMin=[]  DParamMax=[]  NParamMin=[]  NParamMax=[]  KbParamMin=[]  KbParamMax=[]  KtParamMin=[]  KtParamMax=[]  POutMin=[]  POutMax=[]  IOutMin=[]  IOutMax=[]  DOutMin=[]  DOutMax=[]  NOutMin=[]  NOutMax=[]  KbOutMin=[]  KbOutMax=[]  KtOutMin=[]  KtOutMax=[]  IntegratorOutMin=[]  IntegratorOutMax=[]  FilterOutMin=[]  FilterOutMax=[]  SumOutMin=[]  SumOutMax=[]  SumI1OutMin=[]  SumI1OutMax=[]  SumI2OutMin=[]  SumI2OutMax=[]  SumI3OutMin=[]  SumI3OutMax=[]  SumDOutMin=[]  SumDOutMax=[]  SaturationOutMin=[]  SaturationOutMax=[]  IntegratorContinuousStateAttributes=''  IntegratorStateMustResolveToSignalObject=off  IntegratorRTWStateStorageClass=Auto  FilterContinuousStateAttributes=''  FilterStateMustResolveToSignalObject=off  FilterRTWStateStorageClass=Auto
  PID Controller1 : simulink/Continuous/PID Controller  Controller=PI  TimeDomain=Discrete-time  SampleTime=50e-6  IntegratorMethod=Forward Euler  FilterMethod=Forward Euler  Form=Parallel  P=.05  I=.2  D=0  N=100  InitialConditionSource=internal  InitialConditionForIntegrator=0  InitialConditionForFilter=0  ExternalReset=none  LimitOutput=off  UpperSaturationLimit=inf  LowerSaturationLimit=-inf  LinearizeAsGain=on  AntiWindupMode=none  Kb=1  TrackingMode=off  Kt=1  PParamMin=[]  PParamMax=[]  IParamMin=[]  IParamMax=[]  DParamMin=[]  DParamMax=[]  NParamMin=[]  NParamMax=[]  KbParamMin=[]  KbParamMax=[]  KtParamMin=[]  KtParamMax=[]  POutMin=[]  POutMax=[]  IOutMin=[]  IOutMax=[]  DOutMin=[]  DOutMax=[]  NOutMin=[]  NOutMax=[]  KbOutMin=[]  KbOutMax=[]  KtOutMin=[]  KtOutMax=[]  IntegratorOutMin=[]  IntegratorOutMax=[]  FilterOutMin=[]  FilterOutMax=[]  SumOutMin=[]  SumOutMax=[]  SumI1OutMin=[]  SumI1OutMax=[]  SumI2OutMin=[]  SumI2OutMax=[]  SumI3OutMin=[]  SumI3OutMax=[]  SumDOutMin=[]  SumDOutMax=[]  SaturationOutMin=[]  SaturationOutMax=[]  IntegratorContinuousStateAttributes=''  IntegratorStateMustResolveToSignalObject=off  IntegratorRTWStateStorageClass=Auto  FilterContinuousStateAttributes=''  FilterStateMustResolveToSignalObject=off  FilterRTWStateStorageClass=Auto
  Product : Product
  Product1 : Product
  Sum1 : Sum
  i alfa' : Outport  InitialOutput=0
  i beta' : Outport  Port=2  InitialOutput=0
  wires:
  Fcn2/1 -> i alfa'/1
  Fcn3/1 -> i beta'/1
  Product/1 -> Sum1/1
  Product1/1 -> Sum1/2
  Sum1/1 -> PID Controller1/1
  Discrete-Time Integrator/1 -> Fcn1/1, Fcn2/1, Fcn/1, Fcn3/1
  Fcn1/1 -> Product/1
  Fcn/1 -> Product1/2
  vab/1 -> Product/2
  vcb/1 -> Product1/1
  PID Controller/1 -> Integrator/1
  PID Controller1/1 -> Discrete-Time Integrator/1

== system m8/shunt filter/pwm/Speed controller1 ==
  e : Inport
  Discrete-Time Integrator : DiscreteIntegrator  IntegratorMethod=Integration: Backward Euler  SampleTime=50e-6  UpperSaturationLimit=Tlim  LowerSaturationLimit=0  ICPrevOutput=DiscIntNeverNeededParam  ICPrevScaledInput=DiscIntNeverNeededParam
  Gain : Gain  Gain=Ki
  Gain1 : Gain  Gain=Kp
  Sum2 : Sum
  f* : Outport  InitialOutput=0
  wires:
  Gain1/1 -> Sum2/1
  Gain/1 -> Discrete-Time Integrator/1
  e/1 -> Gain/1, Gain1/1
  Discrete-Time Integrator/1 -> Sum2/2
  Sum2/1 -> f*/1

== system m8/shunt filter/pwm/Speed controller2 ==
  e : Inport
  Discrete-Time Integrator : DiscreteIntegrator  IntegratorMethod=Integration: Backward Euler  SampleTime=50e-6  UpperSaturationLimit=Tlim  LowerSaturationLimit=0  ICPrevOutput=DiscIntNeverNeededParam  ICPrevScaledInput=DiscIntNeverNeededParam
  Gain : Gain  Gain=Ki
  Gain1 : Gain  Gain=Kp
  Sum2 : Sum
  f* : Outport  InitialOutput=0
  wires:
  Gain1/1 -> Sum2/1
  Gain/1 -> Discrete-Time Integrator/1
  e/1 -> Gain/1, Gain1/1
  Discrete-Time Integrator/1 -> Sum2/2
  Sum2/1 -> f*/1

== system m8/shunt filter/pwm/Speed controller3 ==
  e : Inport
  Discrete-Time Integrator : DiscreteIntegrator  IntegratorMethod=Integration: Backward Euler  SampleTime=50e-6  UpperSaturationLimit=Tlim  LowerSaturationLimit=0  ICPrevOutput=DiscIntNeverNeededParam  ICPrevScaledInput=DiscIntNeverNeededParam
  Gain : Gain  Gain=Ki
  Gain1 : Gain  Gain=Kp
  Sum2 : Sum
  f* : Outport  InitialOutput=0
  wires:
  Gain1/1 -> Sum2/1
  Gain/1 -> Discrete-Time Integrator/1
  e/1 -> Gain/1, Gain1/1
  Discrete-Time Integrator/1 -> Sum2/2
  Sum2/1 -> f*/1
